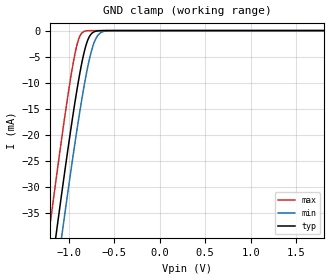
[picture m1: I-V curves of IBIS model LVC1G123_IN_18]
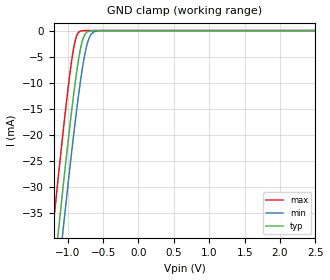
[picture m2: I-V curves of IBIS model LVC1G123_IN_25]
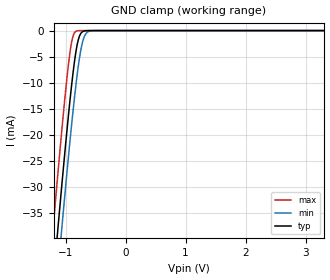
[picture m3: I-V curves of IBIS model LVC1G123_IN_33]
| TEXAS INSTRUMENTS INCORPORATED
| Standard Linear and Logic Group
| IBIS Model of SN74LVC1G123
| SINGLE RETRIGGERABLE MONOSTABLE MULTIVIBRATOR WITH SCHMITT-TRIGGER
| INPUTS
| This file contains package information for the following:
|  TSSOP 8-pin (DCU) package as [Component] LVC1G123_DCU
|  TSSOP 8-pin (DCT) package as [Component] LVC1G123_DCT
|  DSBGA 8-pin (YEP_YZP) package as [Component] LVC1G123_YEP_YZP
| This device can be powered at the following Vccs:
|  1.8 volt Vcc
|  2.5 volt Vcc
|  3.3 volt Vcc
|  5 volt Vcc
| This file provides unique models under the [Model Selector] for each Vcc.
| For operation at a specific Vcc, select the appropriate model after each
| [Model Selector] keyword.
[IBIS Ver]   3.2
[Comment char]  |_char
[File Name]   sn74lvc1g123.ibs
[File Rev]   1.1 | x_die
[Date]   February 17, 2004
[Source]   Data created from TI-SPICE simulations at TI-SLL.
[Notes]   The following is an IBIS list for the LVC1G123.
   Please contact sllibis@ti.com with questions and
   comments concerning SLL IBIS models.
   - FILE REV HISTORY
   - 1.1 Release IBIS file on 04/02/04
   - YEP and YZP packages are package preview only at this date.
   - Power clamp data deleted as there is no power-clamp diode.
   - Due to the fact that the Device is 5.5-V Input tolarent,
   the pulldown model has some Non-Monotonic Warnings.
[Disclaimer] Property of Texas Instruments Incorporated.  Unauthorized
   reproduction and/or distribution is strictly prohibited.
   This product is protected under copyright law.
   Created  2003, (C) Copyright  2003, Texas Instruments
   Incorporated, All Rights Reserved
   UNLESS THERE IS A SIGNED, WRITTEN AGREEMENT TO THE
   CONTRARY, TEXAS INSTRUMENTS (TI) IS PROVIDING THE IBIS
   MODELS  AND WITHOUT ANY WARRANTY, EXPRESSED OR
   IMPLIED.  TI assumes no liability for:
   1) the accuracy of the IBIS models provided to your
   company;
   2) the proper functioning of these IBIS Models in your
   design or for any resulting applications; or
   3) infringement of patents, copyrights or intellectual
   property rights resulting from your use of these IBIS
   models.
   TI provides IBIS Models as a service to our customers.
   You and your company shall not distribute, sell or give
   these models to anyone else without prior written
   permission from TI.
   TI reserves the right to make changes to our products or
   to discontinue any semiconductor product or service
   without notice, and advises our customers to obtain the
   latest version of relevant information to verify, before
   placing orders, that the information being relied on is
   current.
   Please be aware that your receipt and use of the IBIS
   information provided shall serve as acceptance of these
   terms and conditions.  If you do not accept these terms,
   you should return or destroy the IBIS models and any
   other accompanying information immediately.
| Component LVC1G123_DCU 8-pin TSSOP
[Component]   LVC1G123_DCU
[Manufacturer]   Texas Instruments, Inc.
[Package]
|   typ   min   max
R_pkg   1.400e-02   1.300e-02   1.500e-02
L_pkg   1.289e-09   1.025e-09   2.014e-09
C_pkg   1.360e-13   6.600e-14   2.940e-13
[Pin]   signal_name   model_name   R_pin   L_pin   C_pin
1   NA   LVC1G123_IN   1.400e-02   1.387e-09   1.760e-13
2   B   LVC1G123_IN   1.300e-02   1.026e-09   6.600e-14
3   NCLR   LVC1G123_IN   1.300e-02   1.032e-09   6.700e-14
4   GND   GND   1.500e-02   2.014e-09   2.940e-13
5   Q   LVC1G123_OUT   1.400e-02   1.412e-09   1.780e-13
6   CX   LVC1G123_IN   1.300e-02   1.030e-09   6.600e-14
7   RX_CX   LVC1G123_OUT   1.300e-02   1.025e-09   6.600e-14
8   VCC   POWER   1.400e-02   1.386e-09   1.760e-13
| Component LVC1G123_DCT 8-pin TSSOP
[Component]   LVC1G123_DCT
[Manufacturer]   Texas Instruments, Inc.
[Package]
|   typ   min   max
R_pkg   2.900e-02   2.800e-02   3.100e-02
L_pkg   1.796e-09   1.666e-09   1.924e-09
C_pkg   1.090e-13   8.300e-14   1.360e-13
[Pin]   signal_name   model_name   R_pin   L_pin   C_pin
1   NA   LVC1G123_IN   3.100e-02   1.894e-09   1.340e-13
2   B   LVC1G123_IN   2.800e-02   1.697e-09   8.600e-14
3   NCLR   LVC1G123_IN   3.000e-02   1.722e-09   8.600e-14
4   GND   GND   3.000e-02   1.861e-09   1.300e-13
5   Q   LVC1G123_OUT   2.800e-02   1.924e-09   1.360e-13
6   CX   LVC1G123_IN   2.900e-02   1.736e-09   8.600e-14
7   RX_CX   LVC1G123_OUT   2.800e-02   1.666e-09   8.300e-14
8   VCC   POWER   3.000e-02   1.871e-09   1.320e-13
| Component LVC1G123_YEP_YZP 8-pin DSBGA
[Component]   LVC1G123_YEP_YZP
[Manufacturer]   Texas Instruments, Inc.
[Package]
|   typ   min   max
R_pkg   1.000e-03   1.000e-03   4.000e-03
L_pkg   6.400e-11   2.400e-11   3.790e-10
C_pkg   5.800e-14   0.000e+00   6.700e-14
[Pin]   signal_name   model_name   R_pin   L_pin   C_pin
1   NA   LVC1G123_IN   1.000e-03   2.500e-11   6.400e-14
2   B   LVC1G123_IN   1.000e-03   2.400e-11   6.700e-14
3   NCLR   LVC1G123_IN   1.000e-03   2.400e-11   6.700e-14
4   GND   GND   1.000e-03   2.500e-11   6.400e-14
5   Q   LVC1G123_OUT   1.000e-03   2.500e-11   6.400e-14
6   CX   LVC1G123_IN   1.000e-03   2.400e-11   6.700e-14
7   RX_CX   LVC1G123_OUT   1.000e-03   2.400e-11   6.700e-14
8   VCC   POWER   1.000e-03   2.500e-11   6.400e-14
| Model LVC1G123_IN
[Model Selector]   LVC1G123_IN
LVC1G123_IN_18   1.8 volt Vcc
LVC1G123_IN_25   2.5 volt Vcc
LVC1G123_IN_33   3.3 volt Vcc
LVC1G123_IN_50   5 volt Vcc
| Model LVC1G123_OUT
[Model Selector]   LVC1G123_OUT
LVC1G123_OUT_18   1.8 volt Vcc
LVC1G123_OUT_25   2.5 volt Vcc
LVC1G123_OUT_33   3.3 volt Vcc
LVC1G123_OUT_50   5 volt Vcc
| Models and submodels in the file (8): LVC1G123_IN_18 (Input), LVC1G123_IN_25 (Input), LVC1G123_IN_33 (Input), LVC1G123_IN_50 (Input), LVC1G123_OUT_18 (Output), LVC1G123_OUT_25 (Output), LVC1G123_OUT_33 (Output), LVC1G123_OUT_50 (Output)
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[Model]   LVC1G123_IN_18
Model_type  Input
Vinl=0.5775
Vinh=1.2675
| variable   typ   min   max
C_comp   3.10pF   2.61pF   3.77pF
[Temperature Range]   40   100   -40
| Ambient temperature   25   85   -40
[Voltage range]   1.8   1.65   1.95
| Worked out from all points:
|   GND clamp passes 1 mA (typ) near -0.77 V on its own axis
[GND Clamp]
| LVC1G123_IN_18
|   Voltage   I(typ)   I(min)   I(max)
-5.5V     -655.2mA   -662.2mA   -646.6mA
-1.215V   -49.6mA    -57.88mA   -38.96mA
-1.135V   -39.07mA   -47.36mA   -28.42mA
-1.075V   -31.35mA   -39.6mA    -20.75mA
-1.055V   -28.82mA   -37.05mA   -18.27mA
-955mV    -16.68mA   -24.66mA   -6.874mA
-885mV    -9.098mA   -16.55mA   -1.486mA
-825mV    -3.922mA   -10.26mA   -137.1uA
-780mV    -1.472mA   -6.227mA   -17.15uA
-715mV    -205.4uA   -2.128mA   -808.5nA
-650mV    -22.01uA   -443.9uA   -37.93nA
1.8V      3.326pA    6.142pA    3.026pA
[Model]   LVC1G123_IN_25
Model_type  Input
Vinl=0.7
Vinh=1.7
| variable   typ   min   max
C_comp   3.00pF   2.46pF   3.78pF
[Temperature Range]   40   100   -40
| Ambient temperature   25   85   -40
[Voltage range]   2.5   2.3   2.7
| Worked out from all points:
|   GND clamp passes 1 mA (typ) near -0.77 V on its own axis
[GND Clamp]
| LVC1G123_IN_25
|   Voltage   I(typ)   I(min)   I(max)
-5.5V     -655.2mA   -662.2mA   -646.6mA
-1.215V   -49.6mA    -57.88mA   -38.96mA
-1.14V    -39.72mA   -48.01mA   -29.07mA
-1.12V    -37.12mA   -45.41mA   -26.48mA
-1.08V    -31.98mA   -40.25mA   -21.38mA
-1.06V    -29.44mA   -37.69mA   -18.89mA
-960mV    -17.26mA   -25.26mA   -7.377mA
-890mV    -9.597mA   -17.1mA    -1.734mA
-785mV    -1.671mA   -6.635mA   -21.67uA
-720mV    -242.5uA   -2.354mA   -1.023uA
-650mV    -22.01uA   -443.9uA   -37.93nA
2.5V      4.713pA    7.577pA    4.389pA
[Model]   LVC1G123_IN_33
Model_type  Input
Vinl=0.8
Vinh=2.0
| variable   typ   min   max
C_comp   2.91pF   2.35pF   3.80pF
[Temperature Range]   40   100   -40
| Ambient temperature   25   85   -40
[Voltage range]   3.3   3   3.6
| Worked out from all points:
|   GND clamp passes 1 mA (typ) near -0.77 V on its own axis
[GND Clamp]
| LVC1G123_IN_33
|   Voltage   I(typ)   I(min)   I(max)
-5.5V     -655.2mA   -662.2mA   -646.6mA
-1.225V   -50.93mA   -59.21mA   -40.3mA
-1.145V   -40.37mA   -48.66mA   -29.72mA
-1.12V    -37.12mA   -45.41mA   -26.48mA
-1.08V    -31.98mA   -40.25mA   -21.38mA
-1.06V    -29.44mA   -37.69mA   -18.89mA
-965mV    -17.84mA   -25.87mA   -7.89mA
-885mV    -9.098mA   -16.55mA   -1.486mA
-780mV    -1.472mA   -6.227mA   -17.15uA
-715mV    -205.4uA   -2.128mA   -808.5nA
-640mV    -15.53uA   -338.1uA   -23.69nA
3.3V      6.304pA    9.258pA    5.93pA
